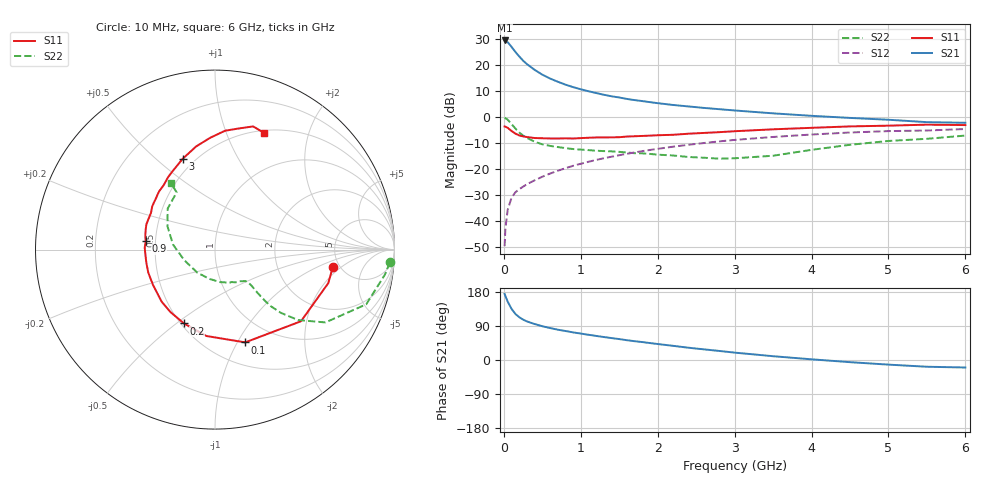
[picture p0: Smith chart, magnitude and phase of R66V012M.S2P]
! SIEMENS Small Signal Semiconductors
! BFR193
! Si NPN RF Bipolar Junction Transistor in SOT23
! VCE = 6 V  IC = 12 mA
! Common Emitter S-Parameters:  May  1996
# GHz  S  MA  R  50
!  f  S11  S21  S12  S22
! GHz  MAG  ANG  MAG  ANG  MAG  ANG  MAG  ANG
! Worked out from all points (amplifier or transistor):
!   36 points, 10 MHz to 6 GHz, reference 50 ohm
!   highest |S21| = 29.5 dB at 10 MHz (marker M1)
!   |S21| within 3 dB of that: start of sweep to 113.9 MHz
!   unconditionally stable (mu >= 1): 701.1 MHz to 2.014 GHz
!   at 250 MHz: K = 0.69, MSG = 24.3 dB, |S12| = -26.7 dB
!   at 1.4 GHz: K = 1.04, MAG = 10.4 dB, |S12| = -15.2 dB
!   at 6 GHz: K = 0.94, MSG = 1.2 dB, |S12| = -4.5 dB
!   S11 on the Smith chart (normalised r, x): 10 MHz: 4.38, -1.54; 100 MHz: 0.73, -1.08; 200 MHz: 0.52, -0.53; 900 MHz: 0.44, +0.05; 3 GHz: 0.43, +0.61; 6 GHz: 0.53, +1.37
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0.01  0.6636 -8.5  29.96 174.4  0.0033 88.2  0.9763 -4.2
0.02  0.6582 -16.5  29.53 168.8  0.0071 83.7  0.9569 -8.4
0.05  0.6236 -39.8  27.77 154.1  0.0165 73.1  0.8959 -19.9
0.1  0.5436 -72.0  22.58 135.0  0.0283 63.7  0.7371 -33.4
0.15  0.4836 -95.7  18.02 121.6  0.0359 58.4  0.6068 -40.3
0.2  0.4463 -112.8  14.76 113.0  0.0411 57.7  0.5097 -43.8
0.25  0.4273 -125.6  12.26 106.6  0.046 57.5  0.4434 -45.4
0.3  0.4154 -135.7  10.51 101.8  0.0513 58.8  0.3995 -45.7
0.4  0.3974 -150.5  8.154 95.0  0.0611 60.4  0.3376 -45.5
0.5  0.3933 -160.8  6.587 89.1  0.0715 62.2  0.3008 -44.9
0.6  0.3895 -168.9  5.559 84.4  0.0822 63.1  0.2807 -44.6
0.7  0.3888 -175.7  4.818 80.1  0.0931 63.9  0.2667 -44.8
0.9  0.3887 173.2  3.792 72.9  0.1161 64.4  0.2439 -45.9
1.1  0.4023 163.6  3.159 66.6  0.1388 64.0  0.2327 -49.3
1.3  0.4077 156.3  2.703 60.6  0.1624 62.8  0.2226 -52.7
1.6  0.4244 145.6  2.246 52.2  0.1977 60.5  0.209 -60.4
2.2  0.4588 128.6  1.719 37.4  0.2707 54.1  0.1834 -81.2
3  0.5371 109.6  1.348 19.5  0.3653 43.3  0.162 -126.9
3.5  0.5847 100.3  1.186 10.0  0.4168 35.8  0.1814 -161.2
4.5  0.6649 85.1  0.969 -5.7  0.5076 21.2  0.2944 154.0
5.5  0.7185 72.8  0.803 -17.8  0.5544 6.2  0.3839 123.8
6  0.7054 67.1  0.781 -19.8  0.5928 1.8  0.4431 123.5
